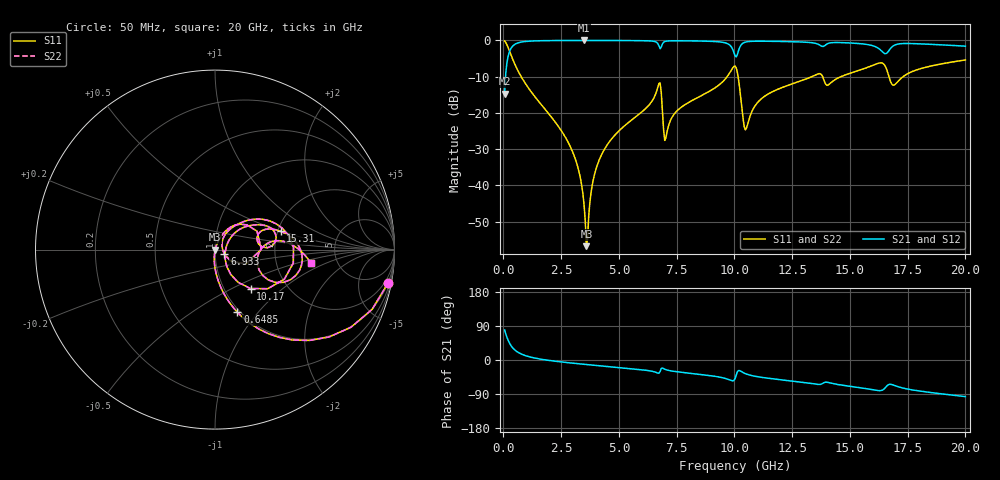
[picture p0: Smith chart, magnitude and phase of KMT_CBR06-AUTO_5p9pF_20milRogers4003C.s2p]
! Data measured by Modelithics Inc. support@modelithics.com 813-866-6335
! KEMET CBR06-AUTO 5.9pF, Pad Width= 0.851mm, Pad Length= 0.64mm, Pad Gap= 0.62mm, 20mil Rogers 4003C substrate Data, January 2022
# hz S ma R 50
! 2 Port Network Data from SP1.SP block
! freq  magS11  angS11  magS21  angS21  magS12  angS12  magS22  angS22
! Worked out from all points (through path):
!   401 points, 50 MHz to 20 GHz, reference 50 ohm
!   highest |S21| = -0.01 dB at 3.491 GHz (marker M1); lowest = -14.7 dB at 50 MHz (marker M2)
!   group delay of S21, straight-line fit = 15 ps
!   lowest |S11| = -56.8 dB at 3.591 GHz (marker M3), VSWR 1.00, Z = 50.1 - j0.104 ohm
!   |S11| at or under -10 dB: 767.7 MHz to 9.685 GHz (8.917 GHz wide, 171 % of centre); 10.16 GHz to 13.35 GHz (3.194 GHz wide, 27.2 % of centre); 13.82 GHz to 14.61 GHz (791.3 MHz wide, 5.57 % of centre)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
!   |S22| runs from -56.8 to -0.1 dB; largest |S21 - S12| = 0
!   S11 on the Smith chart (normalised r, x): 50 MHz: 1, -11; 648.5 MHz: 0.97, -0.79; 6.933 GHz: 1.11, -0.06; 10.17 GHz: 1.32, -0.63; 15.31 GHz: 2.07, +0.49; 20 GHz: 3.18, -0.64
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5e7  0.9829 -10.8  0.1838 79.2  0.1838 79.2  0.9829 -10.8
2.495e8  0.7294 -44.0  0.6835 46.0  0.6835 46.0  0.7294 -44.0
6.485e8  0.371 -70.3  0.928 19.6  0.928 19.6  0.371 -70.3
2.74325e9  0.04255 -95.3  0.9979 -6.7  0.9979 -6.7  0.04255 -95.3
3.391625e9  0.00981 -93.9  0.9987 -10.8  0.9987 -10.8  0.00981 -93.9
3.491375e9  0.005358 -88.6  0.9987 -11.3  0.9987 -11.3  0.005358 -88.6
3.591125e9  0.001449 -46.0  0.9987 -11.9  0.9987 -11.9  0.001449 -46.0
3.94025e9  0.01406 70.9  0.9985 -13.9  0.9985 -13.9  0.01406 70.9
4.289375e9  0.02819 71.4  0.9981 -15.9  0.9981 -15.9  0.02819 71.4
6.73325e9  0.2556 23.6  0.8423 -34.9  0.8423 -34.9  0.2556 23.6
6.93275e9  0.05884 -26.4  0.941 -22.8  0.941 -22.8  0.05884 -26.4
7.0325e9  0.04534 30.5  0.9737 -25.5  0.9737 -25.5  0.04534 30.5
9.626e9  0.2993 34.6  0.9214 -49.0  0.9214 -49.0  0.2993 34.6
1.0025e10  0.4426 -9.8  0.6182 -49.4  0.6182 -49.4  0.4426 -9.8
1.017462e10  0.2938 -47.6  0.7183 -27.8  0.7183 -27.8  0.2938 -47.6
1.052375e10  0.06182 8.5  0.9554 -37.1  0.9554 -37.1  0.06182 8.5
1.127188e10  0.1665 39.9  0.9754 -46.6  0.9754 -46.6  0.1665 39.9
1.336662e10  0.3177 24.3  0.9283 -62.1  0.9283 -62.1  0.3177 24.3
1.531175e10  0.379 15.6  0.9092 -72.0  0.9092 -72.0  0.379 15.6
1.630925e10  0.4896 -7.0  0.7463 -80.9  0.7463 -80.9  0.4896 -7.0
1.670825e10  0.3027 -28.5  0.7381 -64.3  0.7381 -64.3  0.3027 -28.5
2e10  0.5377 -7.7  0.8327 -96.7  0.8327 -96.7  0.5377 -7.7
